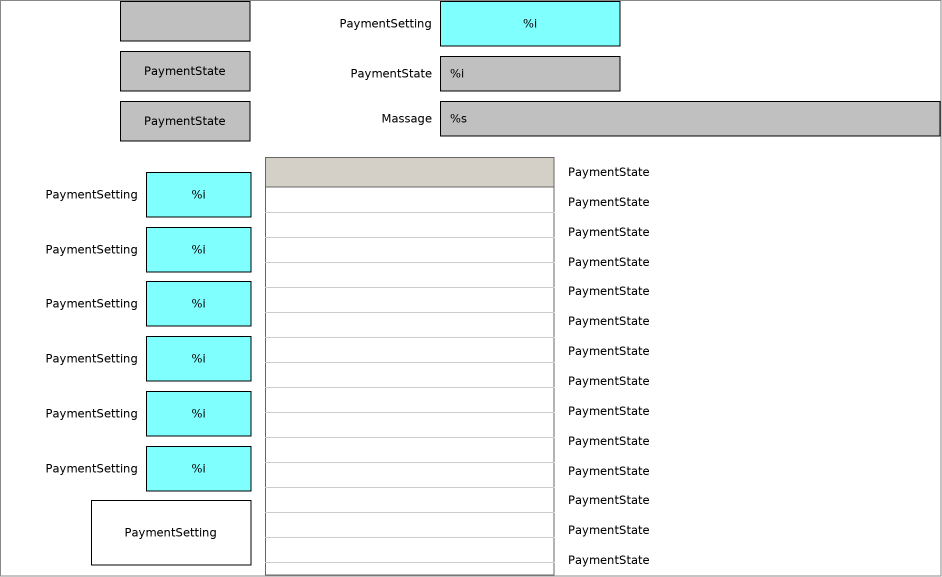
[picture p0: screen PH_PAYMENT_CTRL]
VISUALIZATION PH_PAYMENT_CTRL  // 942x577
VAR_IN_OUT
	fbPaymentDetect			: FB_Payment;	//定义FB的路径
	sPaymentSet_HMI			: ST_Payment	//定义ST的路径
	bSettingInvisible		: BOOL;			//设定参数(年, 月, 日, 密码等)隐藏
	bSettingInputDisable	: BOOL;			//设定参数(年, 月, 日, 密码等)禁止输入
END_VAR
    Rectangle (120,51 130x40), "PaymentState", colour toggle: fbPaymentDetect.bPaymentLock, text list: 'TextList_Payment', text index: 103
    Rectangle (120,101 130x40), "PaymentState", colour toggle: fbPaymentDetect.bPaymentAhead, text list: 'TextList_Payment', text index: 102
    Rectangle (120,1 130x40), colour toggle: fbPaymentDetect.bPaymentEnable, text list: 'TextList_Payment', text index: 100 + BOOL_TO_INT(fbPaymentDetect.bPaymentEnable)
    Rectangle (295,101 140x35), "Massage"
    Rectangle (295,1 140x45), "PaymentSetting", text list: 'TextList_Payment', text index: 9
    Rectangle (440,1 180x45), "%i", text variable: sPaymentSet_HMI.nPassword
        OnMouseClick: write the text variable via VisuDialogs.Numpad
    Rectangle (295,56 140x35), "PaymentState", text list: 'TextList_Payment', text index: 109
    Rectangle (440,56 180x35), "%i", text variable: fbPaymentDetect.nPayLevel
    Rectangle (1,172 140x45), "PaymentSetting", text list: 'TextList_Payment', text index: 1
    Rectangle (1,227 140x45), "PaymentSetting", text list: 'TextList_Payment', text index: 2
    Rectangle (1,281 140x45), "PaymentSetting", text list: 'TextList_Payment', text index: 3
    Rectangle (1,336 140x45), "PaymentSetting", text list: 'TextList_Payment', text index: 4
    Rectangle (1,391 140x45), "PaymentSetting", text list: 'TextList_Payment', text index: 5
    Rectangle (1,446 140x45), "PaymentSetting", text list: 'TextList_Payment', text index: 6
    Group (91,157 833x418), invisible if: bSettingInvisible, input disabled if: bSettingInputDisable
        Rectangle (0,343 160x65), "PaymentSetting", colour toggle: sPaymentSet_HMI.bEnable, text list: 'TextList_Payment', text index: 0
            tap sPaymentSet_HMI.bEnable
        Table (174,0 289x418), data array: sPaymentSet_HMI.anPaymentPassword
            p3854506369: sPaymentSet_HMI.anPaymentPassword[INDEX]
            Columns.Column.[0].Template: sPaymentSet_HMI.anPaymentPassword[INDEX] <> 0; OnMouseClick: write the text variable via VisuDialogs.Numpad
        Rectangle (55,15 105x45), "%i", text variable: sPaymentSet_HMI.wYear, colour toggle: fbPaymentDetect.bPaymentEnable, input disabled if: fbPaymentDetect.bPaymentEnable
            OnMouseClick: write the text variable via VisuDialogs.Numpad
        Rectangle (55,70 105x45), "%i", text variable: sPaymentSet_HMI.wMonth, colour toggle: fbPaymentDetect.bPaymentEnable, input disabled if: fbPaymentDetect.bPaymentEnable
            OnMouseClick: write the text variable via VisuDialogs.Numpad
        Rectangle (55,124 105x45), "%i", text variable: sPaymentSet_HMI.wDay, colour toggle: fbPaymentDetect.bPaymentEnable, input disabled if: fbPaymentDetect.bPaymentEnable
            OnMouseClick: write the text variable via VisuDialogs.Numpad
        Rectangle (55,179 105x45), "%i", text variable: sPaymentSet_HMI.iPaymentNo, colour toggle: fbPaymentDetect.bPaymentEnable, input disabled if: fbPaymentDetect.bPaymentEnable
            OnMouseClick: write the text variable via VisuDialogs.Numpad
        Rectangle (55,234 105x45), "%i", text variable: sPaymentSet_HMI.iMonth, colour toggle: fbPaymentDetect.bPaymentEnable, input disabled if: fbPaymentDetect.bPaymentEnable
            OnMouseClick: write the text variable via VisuDialogs.Numpad
        Rectangle (55,289 105x45), "%i", text variable: sPaymentSet_HMI.iAheadDays, colour toggle: fbPaymentDetect.bPaymentEnable, input disabled if: fbPaymentDetect.bPaymentEnable
            OnMouseClick: write the text variable via VisuDialogs.Numpad
        Rectangle (474,0 359x30), "PaymentState", text list: 'TextList_Payment', text index: 110
        Rectangle (474,30 359x30), "PaymentState", text list: 'TextList_Payment', text index: 111
        Rectangle (474,60 359x30), "PaymentState", text list: 'TextList_Payment', text index: 112
        Rectangle (474,90 359x30), "PaymentState", text list: 'TextList_Payment', text index: 113
        Rectangle (474,119 359x30), "PaymentState", text list: 'TextList_Payment', text index: 114
        Rectangle (474,149 359x30), "PaymentState", text list: 'TextList_Payment', text index: 115
        Rectangle (474,179 359x30), "PaymentState", text list: 'TextList_Payment', text index: 116
        Rectangle (474,209 359x30), "PaymentState", text list: 'TextList_Payment', text index: 117
        Rectangle (474,239 359x30), "PaymentState", text list: 'TextList_Payment', text index: 118
        Rectangle (474,269 359x30), "PaymentState", text list: 'TextList_Payment', text index: 119
        Rectangle (474,299 359x30), "PaymentState", text list: 'TextList_Payment', text index: 120
        Rectangle (474,328 359x30), "PaymentState", text list: 'TextList_Payment', text index: 121
        Rectangle (474,358 359x30), "PaymentState", text list: 'TextList_Payment', text index: 122
        Rectangle (474,388 359x30), "PaymentState", text list: 'TextList_Payment', text index: 123
    Rectangle (440,101 500x35), "%s", text variable: sPaymentSet_HMI.sgMassage
END_VISUALIZATION
